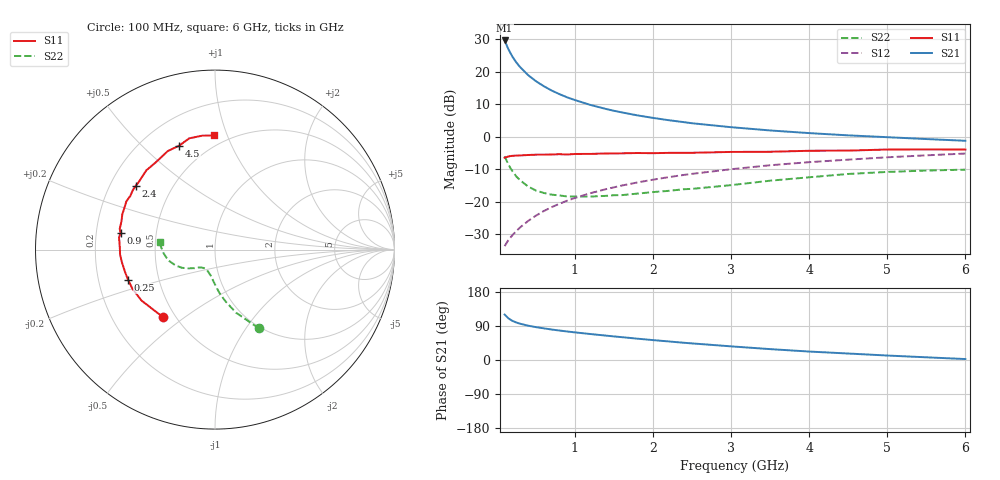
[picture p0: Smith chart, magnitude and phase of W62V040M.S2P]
! SIEMENS Small Signal Semiconductors
! BFR193W
! Si NPN RF Bipolar Junction Transistor in SOT323
! VCE = 2 V  IC = 40 mA
! Common Emitter S-Parameters:  September  1992
# GHz  S  MA  R  50
!  f  S11  S21  S12  S22
! GHz  MAG  ANG  MAG  ANG  MAG  ANG  MAG  ANG
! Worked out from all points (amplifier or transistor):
!   28 points, 100 MHz to 6 GHz, reference 50 ohm
!   highest |S21| = 29.7 dB at 100 MHz (marker M1)
!   |S21| within 3 dB of that: start of sweep to 154.8 MHz
!   unconditionally stable (mu >= 1): 508.7 MHz to 2.539 GHz
!   at 300 MHz: K = 0.91, MSG = 24.7 dB, |S12| = -27.9 dB
!   at 1.5 GHz: K = 1.04, MAG = 10.6 dB, |S12| = -15.6 dB
!   at 6 GHz: K = 0.93, MSG = 2.0 dB, |S12| = -5.2 dB
!   S11 on the Smith chart (normalised r, x): 100 MHz: 0.43, -0.42; 250 MHz: 0.33, -0.15; 900 MHz: 0.31, +0.08; 2.4 GHz: 0.31, +0.32; 4.5 GHz: 0.35, +0.65; 6 GHz: 0.42, +0.90
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0.1  0.4749 -127.8  30.55 120.0  0.0206 59.1  0.5022 -60.9
0.15  0.4982 -145.2  22.16 109.7  0.0258 60.0  0.3698 -71.6
0.2  0.509 -154.5  17.21 103.2  0.0304 62.0  0.2945 -78.5
0.25  0.5128 -160.9  14.01 99.0  0.0353 64.2  0.2443 -84.0
0.3  0.5162 -165.7  11.82 95.6  0.0402 65.9  0.2131 -87.5
0.4  0.5239 -172.5  8.952 90.6  0.0503 68.8  0.1716 -93.8
0.5  0.5296 -177.1  7.213 86.8  0.0608 70.2  0.1486 -98.6
0.6  0.5303 179.0  6.042 83.6  0.0715 71.0  0.1363 -103.7
0.7  0.5335 175.9  5.177 80.5  0.082 71.5  0.1285 -107.0
0.8  0.5392 172.8  4.558 77.8  0.0926 71.6  0.1247 -110.3
0.9  0.5336 170.2  4.06 75.3  0.1034 71.5  0.1204 -113.0
1  0.5434 167.7  3.683 72.9  0.114 71.2  0.12 -115.3
1.2  0.5446 162.9  3.095 68.5  0.1352 70.3  0.1199 -121.1
1.4  0.5531 159.0  2.68 64.3  0.1561 69.3  0.1229 -124.7
1.6  0.5563 154.9  2.379 60.3  0.1771 68.1  0.1261 -128.5
1.8  0.5622 151.5  2.139 56.3  0.1976 66.6  0.1331 -131.6
2.2  0.5653 144.1  1.803 49.0  0.2386 63.6  0.1468 -135.7
2.4  0.5668 141.0  1.679 45.4  0.2588 61.9  0.1556 -138.2
3.5  0.5877 124.1  1.252 28.7  0.3642 52.3  0.2106 -151.2
4.5  0.6128 108.9  1.052 17.1  0.4445 43.2  0.2674 -167.2
5.5  0.6387 96.5  0.923 7.1  0.5178 34.5  0.3018 176.9
6  0.6361 90.3  0.868 2.5  0.5519 29.9  0.3116 172.1
